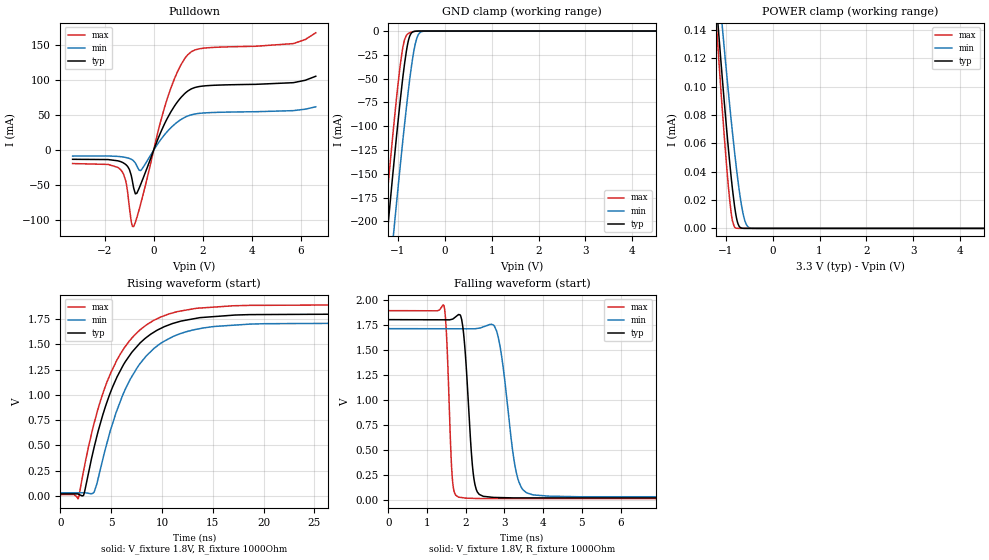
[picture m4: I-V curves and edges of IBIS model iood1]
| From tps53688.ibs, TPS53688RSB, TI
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|   iood1 Model
[Model]   iood1
Model_type   I/O_open_drain
Polarity   Non-Inverting
Enable   Active-Low
Vinl = 0.95
Vinh = 1.2
Vmeas = 0.9
Vref = 1.8
Cref = 2pF
Rref = 1000
|   typ   min   max
C_comp   1.498pF   1.478pF   1.533pF
[Voltage Range]   3.3   2.95   3.6
[Temperature Range]   25   125   -40
[Pullup Reference]   3.3   2.95   3.6
[Pulldown Reference]   0   0   0
[Power Clamp Reference]   3.3   2.95   3.6
[GND Clamp Reference]   0   0   0
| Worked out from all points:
|   slope of the pulldown table from 0 to 0.495 V, typ, clamps not added: 12 ohm
|   GND clamp passes 1 mA (typ) near -0.68 V on its own axis
|   falling waveform, V_fixture 1.8V, R_fixture 1000Ohm: 20-80 % time 173ps typ, 311ps min, 107ps max; typ from 1.8 V to 0.018 V
|   rising waveform, V_fixture 1.8V, R_fixture 1000Ohm: 20-80 % time 4.15ns typ, 4.18ns min, 4.09ns max; typ from 0.018 V to 1.8 V
[Pulldown]
|   Voltage   I(typ)   I(min)   I(max)
-3.3V     -13.02mA   -8.374mA   -19.12mA
-1.36V    -16.18mA   -9.206mA   -27.37mA
-1.142V   -20.33mA   -10.35mA   -43.19mA
-914.1mV  -35.89mA   -12.87mA   -101.8mA
-815.1mV  -53.99mA   -15.31mA   -109.3mA
-686.4mV  -61.62mA   -22.22mA   -96.74mA
-518.1mV  -48.03mA   -28.74mA   -75.45mA
511.5mV   42.56mA    25.04mA    69.09mA
937.2mV   67.68mA    39.52mA    109.7mA
1.393V    84.74mA    49.01mA    136.7mA
5.679V    96.61mA    56.61mA    152.5mA
6.6V      105.8mA    62.11mA    168mA
[GND Clamp]
|   Voltage   I(typ)   I(min)   I(max)
-3.3V     -1.405A    -1.453A    -1.382A
-1.29V    -249mA     -319mA     -208.3mA
-1.201V   -201mA     -271.5mA   -159.8mA
-1.102V   -149.1mA   -219.8mA   -107.8mA
-1.033V   -114.1mA   -184.4mA   -73.6mA
-894.3mV  -49.89mA   -116.3mA   -18.01mA
-815.1mV  -20.86mA   -80.11mA   -4.459mA
-735.9mV  -4.319mA   -47.36mA   -1.626mA
-666.6mV  -668.5uA   -23.79mA   -584.8uA
-597.3mV  -117.1uA   -8.141mA   -142.1uA
-468.6mV  -4.717uA   -333.4uA   -4.309uA
6.6V      0A         0A         0A
[POWER Clamp]
|   Voltage   I(typ)   I(min)   I(max)
-3.3V     1.121mA    1.045mA    1.255mA
-1.191V   155.6uA    186.9uA    140.7uA
-1.082V   110.3uA    146.1uA    88.65uA
-1.033V   90.47uA    128.1uA    66.34uA
-943.8mV  56.9uA     96.84uA    30.13uA
-884.4mV  36.69uA    77uA       11.39uA
-854.7mV  27.56uA    67.48uA    5.149uA
-785.4mV  10.26uA    46.56uA    269.6nA
-716.1mV  1.685uA    28.1uA     0A
-617.1mV  27.6nA     8.619uA    0A
-468.6mV  0A         239.7nA    0A
6.6V      0A         0A         0A
[Ramp]
R_load = 1000
|   typ   min   max
dV/dt_r   1.06894/4.14042e-09   1.00831/4.1817e-09   1.12685/4.09105e-09
dV/dt_f   1.06894/1.73353e-10   1.00831/3.11362e-10   1.12685/1.07199e-10
[Falling Waveform]
V_fixture = 1.8V
V_fixture_min = 1.71V
V_fixture_max = 1.89V
R_fixture = 1000Ohm
C_fixture = 0F
|   Time   V(typ)   V(min)   V(max)
0s        1.8V       1.71V      1.89V
1.432ns   1.798V     1.709V     1.943V
1.66ns    1.805V     1.709V     186.7mV
1.857ns   1.847V     1.709V     25.24mV
2.189ns   278.2mV    1.708V     15.2mV
2.394ns   46.63mV    1.719V     12.88mV
2.816ns   23.86mV    1.661V     12.88mV
3.428ns   19.72mV    130.7mV    12.88mV
4.927ns   19.71mV    31.28mV    12.88mV
500ns     18.44mV    29.49mV    11.92mV
[Rising Waveform]
V_fixture = 1.8V
V_fixture_min = 1.71V
V_fixture_max = 1.89V
R_fixture = 1000Ohm
C_fixture = 0F
|   Time   V(typ)   V(min)   V(max)
0s        18.44mV    29.49mV    11.92mV
1.756ns   16.56mV    29.86mV    -26.4mV
2.284ns   6.955mV    29.97mV    249.8mV
3.318ns   481.3mV    36.72mV    719.2mV
5.158ns   1.083V     723mV      1.26V
7.275ns   1.449V     1.221V     1.589V
9.217ns   1.621V     1.46V      1.738V
11.11ns   1.708V     1.578V     1.813V
17.02ns   1.789V     1.689V     1.882V
500ns     1.8V       1.71V      1.89V
